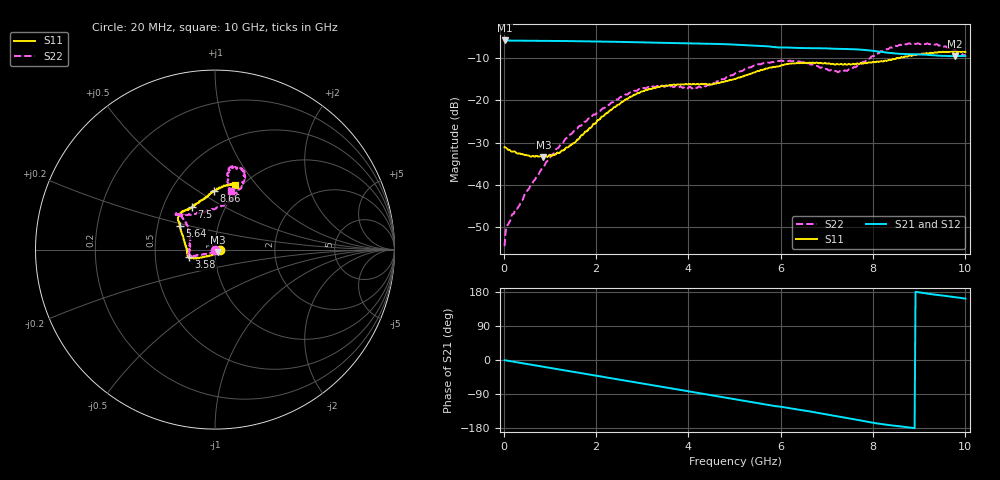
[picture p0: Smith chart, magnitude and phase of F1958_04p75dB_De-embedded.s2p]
! Integrated Device Technology
! Corporate Headquarters
! 6024 Silver Creek Valley Road
! San Jose, CA 95138  USA
! Phone:  1-408-284-8200
! Toll Free:  1-800-223-1366
! Webpage:  http://www.idt.com/
! Timing and RF Division
! 515 Groton Road, Suite 102
! Westford, MA 01886-6024
! Device:  F1958
! Description: 7-bit 0.25 dB Digital Step Attenuator
! Frequency:  0.001 -  6.000 GHz
! Package:  4x4 mm Thin QFN Plastic Package: 24 pin
! Ports:  2 RF, 12 DC
!  Pin  1  = D0
!  Pin  2  = VDD
!  Pin  3  = VMODE
!  Pin  4  = GND
!  Pin  5  = RF1  =  Port 1
!  Pin  6  = GND
!  Pin  7  = GND
!  Pin  8  = GND
!  Pin  9  = GND
!  Pin 10  = GND
!  Pin 11  = GND
!  Pin 12  = GND
!  Pin 13  = GND
!  Pin 14  = RF2  =  Port 2
!  Pin 15  = GND
!  Pin 16  = LE
!  Pin 17  = CLK
!  Pin 18  = DATA
!  Pin 19  = D6
!  Pin 20  = D5
!  Pin 21  = D4
!  Pin 22  = D3
!  Pin 23  = D2
!  Pin 24  = D1
! State:  19
! Atten State:  4.75 dB
! Voltage:  +3.30 Volts
! Current:  0.258 mA
! Data:  The device was measured on a F1958 evaluation board which has
!  individual transmission lines to the RF pins.  Data was collected
!  using a calibrated network analyzer.  The evaluation board was
!  de-embedded using Automatic Fixture Removal (AFR).
!  The reference plane is the edge of the package pin.
! Misc:
!  Action Tracker AT0419
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# GHz S dB R 50
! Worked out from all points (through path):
!   500 points, 20 MHz to 10 GHz, reference 50 ohm
!   highest |S21| = -5.77 dB at 20 MHz (marker M1); lowest = -9.5 dB at 9.78 GHz (marker M2)
!   group delay of S21, straight-line fit = 56.1 ps
!   lowest |S11| = -33.5 dB at 860 MHz (marker M3), VSWR 1.04, Z = 51.4 - j1.63 ohm
!   |S11| at or under -10 dB: start of sweep to 8.509 GHz
!   |S22| runs from -54.6 to -6.4 dB; largest |S21 - S12| = 0.0015
!   S11 on the Smith chart (normalised r, x): 20 MHz: 1.06, -0.00; 3.58 GHz: 0.74, -0.07; 5.64 GHz: 0.65, +0.18; 7.5 GHz: 0.70, +0.35; 8.66 GHz: 0.80, +0.58; 10 GHz: 0.94, +0.78
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0.02  -31.10 -4.3  -5.77 -0.6  -5.77 -0.5  -54.56 -75.4
0.08  -31.59 -7.6  -5.79 -1.8  -5.79 -1.8  -49.59 -93.5
0.22  -32.08 -13.4  -5.81 -4.7  -5.81 -4.7  -46.86 -113.1
0.86  -33.47 -48.3  -5.86 -17.8  -5.85 -17.8  -35.84 -132.4
1.24  -32.08 -87.3  -5.89 -25.7  -5.89 -25.7  -30.24 -142.3
1.7  -28.20 -122.0  -5.96 -35.1  -5.95 -35.1  -25.65 -153.6
2.6  -20.16 -152.0  -6.13 -53.7  -6.11 -53.7  -18.92 -163.0
2.94  -18.18 -156.8  -6.20 -60.7  -6.19 -60.8  -17.29 -163.7
3.36  -16.79 -160.8  -6.31 -69.3  -6.31 -69.4  -16.70 -166.8
3.58  -16.41 -163.3  -6.35 -73.8  -6.35 -73.9  -16.79 -171.2
4.3  -16.07 -174.4  -6.49 -88.7  -6.51 -88.7  -16.72 162.1
5.02  -14.89 162.9  -6.74 -103.8  -6.75 -103.8  -13.53 138.9
5.64  -12.62 146.4  -7.10 -116.7  -7.11 -116.7  -11.20 135.8
6.16  -11.33 139.2  -7.44 -126.5  -7.46 -126.4  -10.66 137.4
6.68  -11.04 132.0  -7.60 -136.7  -7.62 -136.6  -11.48 132.6
7.2  -11.42 123.6  -7.74 -147.7  -7.75 -147.5  -13.01 108.5
7.5  -11.41 118.8  -7.84 -154.3  -7.84 -154.2  -12.56 87.5
8.34  -10.40 98.0  -8.70 -171.7  -8.70 -171.8  -7.72 66.9
8.66  -9.76 90.7  -8.98 -176.1  -8.99 -176.1  -6.64 69.2
9.3  -8.73 78.0  -9.26 173.1  -9.27 173.1  -6.63 79.7
9.78  -8.40 73.8  -9.50 165.9  -9.53 165.9  -8.05 79.3
10  -8.51 72.7  -9.44 161.9  -9.47 162.0  -9.45 74.8
